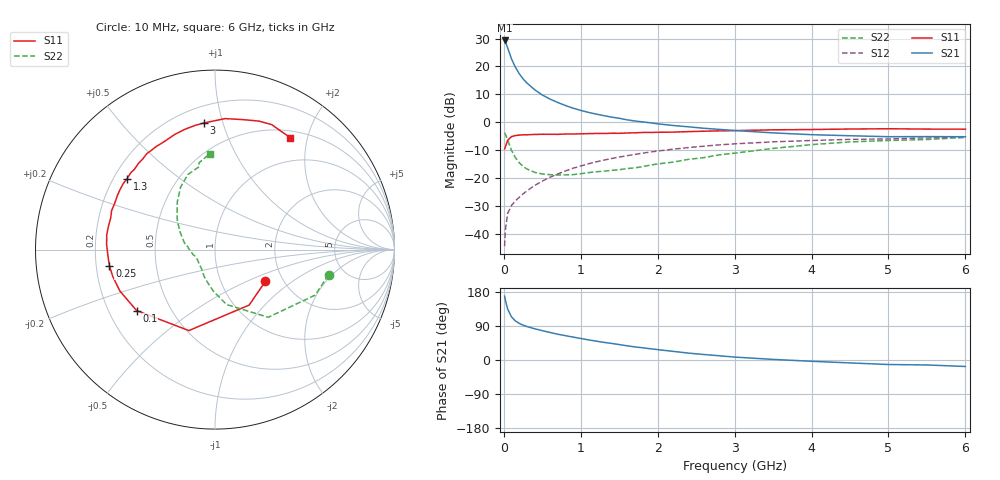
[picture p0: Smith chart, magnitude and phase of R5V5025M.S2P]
! SIEMENS Small Signal Semiconductors
! BFR183
! Si NPN RF Bipolar Junction Transistor in SOT23
! VCE = 0.5 V  IC = 25 mA
! Common Emitter S-Parameters:  May  1996
# GHz  S  MA  R  50
!  f  S11  S21  S12  S22
! GHz  MAG  ANG  MAG  ANG  MAG  ANG  MAG  ANG
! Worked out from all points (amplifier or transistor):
!   36 points, 10 MHz to 6 GHz, reference 50 ohm
!   highest |S21| = 29.3 dB at 10 MHz (marker M1)
!   |S21| within 3 dB of that: start of sweep to 53.8 MHz
!   unconditionally stable (mu >= 1): start of sweep to 16.36 MHz; 177.7 MHz to end of sweep
!   at 250 MHz: K = 1.14, MAG = 18.4 dB, |S12| = -25.7 dB
!   at 1.4 GHz: K = 1.26, MAG = 4.3 dB, |S12| = -13.0 dB
!   at 6 GHz: K = 1.07, MAG = -1.6 dB, |S12| = -5.4 dB
!   S11 on the Smith chart (normalised r, x): 10 MHz: 1.62, -0.64; 100 MHz: 0.32, -0.31; 250 MHz: 0.26, -0.07; 1.3 GHz: 0.25, +0.33; 3 GHz: 0.31, +0.87; 6 GHz: 0.60, +1.72
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0.01  0.3319 -32.2  29.31 168.5  0.006 74.2  0.6485 -12.5
0.02  0.3629 -58.4  27.85 157.9  0.0119 71.0  0.6132 -24.4
0.05  0.4741 -107.9  21.47 134.1  0.0232 58.4  0.4798 -51.8
0.1  0.5533 -142.1  13.66 113.6  0.0323 52.5  0.3132 -78.0
0.15  0.5781 -156.5  9.703 103.1  0.0389 53.6  0.2328 -92.0
0.2  0.5891 -165.4  7.434 96.6  0.0451 56.1  0.1879 -102.7
0.25  0.5951 -171.3  5.995 91.9  0.052 58.7  0.1617 -112.0
0.3  0.5966 -175.6  5.06 88.3  0.0588 60.6  0.1455 -117.5
0.4  0.6046 177.3  3.839 82.5  0.0735 62.9  0.1265 -128.2
0.5  0.609 172.2  3.085 77.4  0.0881 64.0  0.1184 -138.3
0.6  0.6077 167.5  2.607 72.7  0.1035 64.2  0.115 -144.7
0.7  0.6071 163.2  2.265 68.0  0.1184 64.0  0.1133 -149.3
0.9  0.6154 155.3  1.789 60.4  0.1498 62.5  0.1152 -159.4
1.1  0.6258 147.9  1.504 53.1  0.1799 60.1  0.125 -166.8
1.3  0.6293 141.0  1.313 46.5  0.2093 57.3  0.1327 -174.2
1.7  0.6461 128.4  1.055 34.6  0.2645 51.2  0.1518 173.8
2.2  0.6658 114.6  0.876 22.8  0.329 42.8  0.1929 160.6
3  0.7081 95.0  0.712 7.7  0.4104 28.9  0.2792 139.1
3.5  0.7321 85.6  0.645 1.6  0.4457 20.7  0.3396 128.2
4.5  0.7564 71.2  0.573 -7.7  0.4934 6.6  0.4447 109.9
5.5  0.7545 60.3  0.553 -13.1  0.5262 -3.7  0.491 100.5
6  0.7519 56.0  0.55 -17.1  0.5383 -10.6  0.5351 93.2
